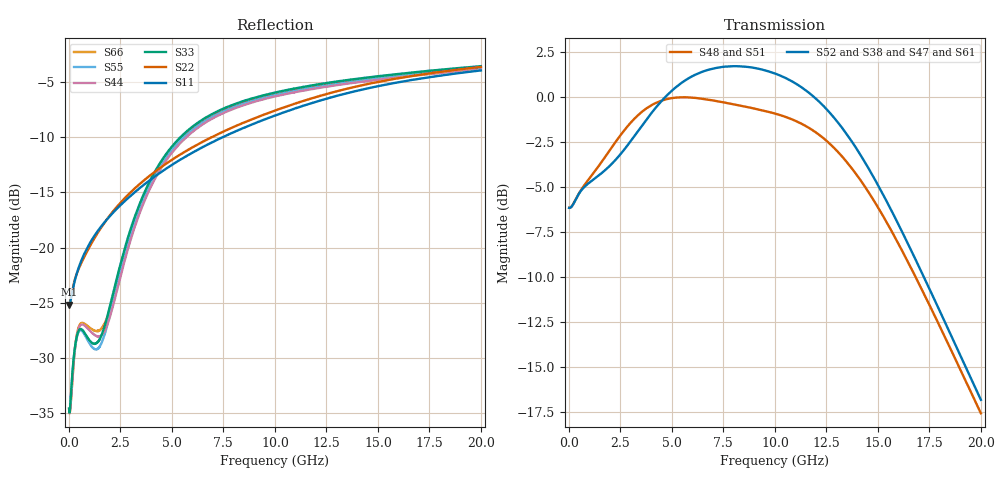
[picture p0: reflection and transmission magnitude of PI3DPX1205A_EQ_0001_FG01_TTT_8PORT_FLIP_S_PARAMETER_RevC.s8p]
! NPort=8 DATA=2000 NOISE=0 GROUPDELAY=0 COMPLEX_DATAFORMAT=POLAR
! NumOfBlock=1 NumOfParam=0
! .MODEL Smodel S TSTONEFILE=PI3DPX1205A_EQ_0001_FG01_TTT_8PORT_FLIP_S_PARAMETER_RevC.s8p TYPE=S
!  -- The above .MODEL line can be used for the S element in the netlist.
! The s parameter is extracted from the linear redriver, it is not bi-directional;
! only s(5,1)s(6,2)s(3,7)s(4,8) should be the insertion loss
!  Port definition:
!  Port1 = AIP
!  Port2 = AIN
!  Port3 = BOP
!  Port4 = BON
!  Port5 = AOP
!  Port6 = AON
!  Port7 = BIP
!  Port8 = BIN
# Hz S MA R  50
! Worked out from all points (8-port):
!   2000 points, 10 MHz to 20 GHz, reference 50 ohm
!   strongest paths, dB at 10 MHz, 5.01 GHz, 10.01 GHz, 15.01 GHz, 20 GHz:
!     S52: -6.1, 0.4, 1.3, -4.9, -16.8
!     S38: -6.1, 0.4, 1.3, -4.9, -16.8
!     S47: -6.1, 0.4, 1.3, -4.9, -16.8
!     S61: -6.1, 0.3, 1.3, -4.9, -16.8
!     S48: -6.1, 0.0, -0.9, -6.1, -17.6
!     S51: -6.1, -0.1, -0.9, -6.2, -17.6
!   lowest |S11| = -25.2 dB at 10 MHz (marker M1), VSWR 1.12, Z = 44.8 - j0.115 ohm
!   |S11| at or under -10 dB: start of sweep to 7.47 GHz
